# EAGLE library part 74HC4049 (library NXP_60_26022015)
Hex inverting HIGH-to-LOW level shifter The 74HC4049 is a hex inverter with over-voltage tolerant inputs. Inputs are overvoltage tolerant to 15 V. This enables the device to be used in HIGH-to-LOW level shifting applications. AAL Eindhoven MK
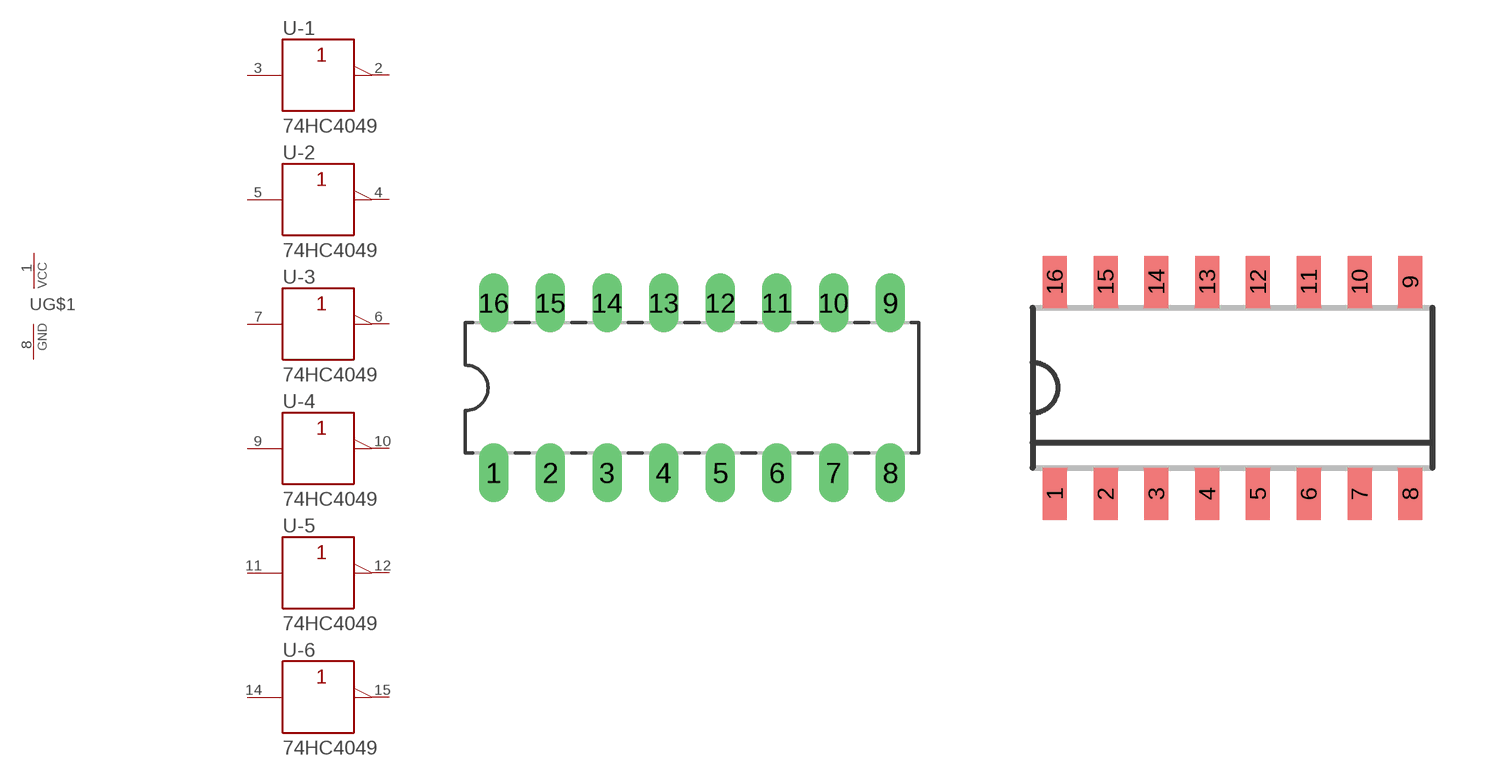
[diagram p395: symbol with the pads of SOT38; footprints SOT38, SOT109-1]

Designator prefix U; gates -1=INVERTER -2=INVERTER -3=INVERTER -4=INVERTER -5=INVERTER -6=INVERTER G$1=PWRN

## 74HC4049N  [SOT38]
1  G$1:VCC  pwr
2  -1:Y  out
3  -1:A  in
4  -2:Y  out
5  -2:A  in
6  -3:Y  out
7  -3:A  in
8  G$1:GND  pwr
9  -4:A  in
10  -4:Y  out
11  -5:A  in
12  -5:Y  out
14  -6:A  in
15  -6:Y  out

## 74HC4049D  [SOT109-1]
Pads as for SOT38

## 74HC4049DB  [SOT338]
Pads as for SOT38

## 74HC4049PW  [SOT403-1]
Pads as for SOT38

## Footprint SOT38 (pad centres in mm)
Dual In Line Package
drill 0.813 long: 1 -8.89,-3.81; 2 -6.35,-3.81; 3 -3.81,-3.81; 4 -1.27,-3.81; 5 1.27,-3.81; 6 3.81,-3.81; 7 6.35,-3.81; 8 8.89,-3.81; 9 8.89,3.81; 10 6.35,3.81; 11 3.81,3.81; 12 1.27,3.81; 13 -1.27,3.81; 14 -3.81,3.81; 15 -6.35,3.81; 16 -8.89,3.81

## Footprint SOT109-1 (pad centres in mm)
SOT109-1 SO16: plastic small outline package; 16 leads; body width 3.9 mm JEDEC: MS-012 IEC: 076E07
smd 0.6 x 1.3: 1 -4.445,-2.65; 2 -3.175,-2.65; 3 -1.905,-2.65; 4 -0.635,-2.65; 5 0.635,-2.65; 6 1.905,-2.65; 7 3.175,-2.65; 8 4.445,-2.65; 9 4.445,2.65; 10 3.175,2.65; 11 1.905,2.65; 12 0.635,2.65; 13 -0.635,2.65; 14 -1.905,2.65; 15 -3.175,2.65; 16 -4.445,2.65

## Footprint SOT338 (pad centres in mm)
SOT338 SSOP16: plastic shrink small outline package; 16 leads; body width 5.3 mm JEDEC: MO-150 IEC: --
smd 0.4 x 1.2: 1 -2.275,-3.45; 2 -1.625,-3.45; 3 -0.975,-3.45; 4 -0.325,-3.45; 5 0.325,-3.45; 6 0.975,-3.45; 7 1.625,-3.45; 8 2.275,-3.45; 9 2.275,3.45; 10 1.625,3.45; 11 0.975,3.45; 12 0.325,3.45; 13 -0.325,3.45; 14 -0.975,3.45; 15 -1.625,3.45; 16 -2.275,3.45

## Footprint SOT403-1 (pad centres in mm)
SOT403-1 TSSOP16: plastic thin shrink small outline package; 16 leads; body width 4.4 mm JEDEC: MO-153 IEC: ---
smd 0.6 x 1.35: 1 -2.375,-2.925; 8 2.375,-2.925; 9 2.375,2.925; 16 -2.375,2.925
smd 0.4 x 1.35: 2 -1.625,-2.925; 3 -0.975,-2.925; 4 -0.325,-2.925; 5 0.325,-2.925; 6 0.975,-2.925; 7 1.625,-2.925; 10 1.625,2.925; 11 0.975,2.925; 12 0.325,2.925; 13 -0.325,2.925; 14 -0.975,2.925; 15 -1.625,2.925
